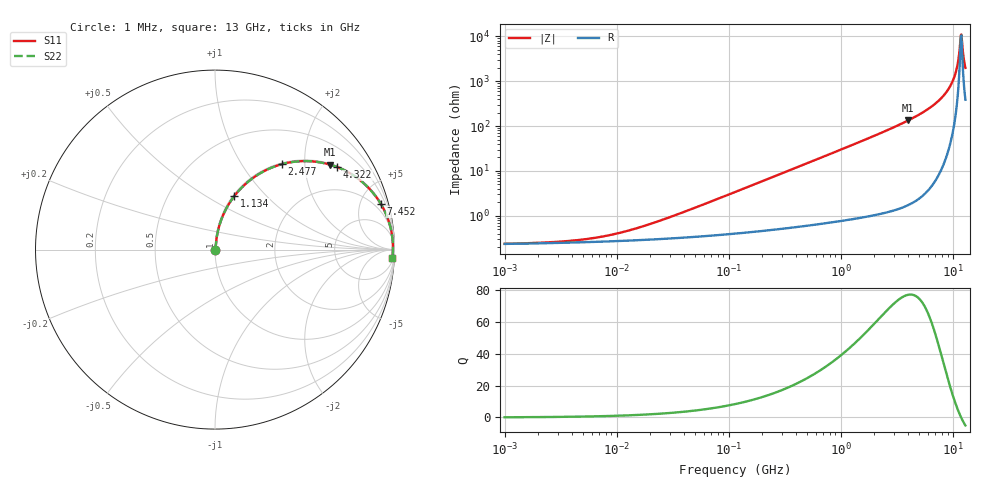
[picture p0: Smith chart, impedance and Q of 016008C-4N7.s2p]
# MHz S MA R 50
!Freq  MagS11  AngS11  MagS21  AngS21  MagS12  AngS12  MagS22  AngS22
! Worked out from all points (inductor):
!   801 points, 1 MHz to 13 GHz, reference 50 ohm
!   read as one part in series: L = 4.7 nH near 32.5 MHz
!   highest Q = 76.9 at 4.026 GHz (marker M1), where L = 5.31 nH
!   self-resonance near 11.83 GHz
!   S11 on the Smith chart (normalised r, x): 1 MHz: 1.00, +0.00; 1.134 GHz: 1.02, +0.68; 2.477 GHz: 1.02, +1.53; 4.322 GHz: 1.04, +2.94; 7.452 GHz: 1.16, +7.23; 13 GHz: 9, -39
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1  0.002383 7.1  0.9976 -0.0  0.9976 -0.0  0.002383 7.1
4.887486  0.002945 29.2  0.9974 -0.1  0.9974 -0.1  0.002945 29.2
10.428  0.004117 48.1  0.9973 -0.2  0.9973 -0.2  0.004117 48.1
23.60634  0.007577 66.1  0.997 -0.4  0.997 -0.4  0.007577 66.1
114.0175  0.03376 81.3  0.9954 -1.9  0.9954 -1.9  0.03376 81.3
557.2591  0.1619 78.5  0.9807 -9.3  0.9807 -9.3  0.1619 78.5
1133.974  0.3179 70.1  0.9406 -18.5  0.9406 -18.5  0.3179 70.1
1696.077  0.4519 62.1  0.8837 -26.9  0.8837 -26.9  0.4519 62.1
2477.441  0.6031 52.0  0.7886 -37.1  0.7886 -37.1  0.6031 52.0
2691.536  0.6376 49.6  0.7611 -39.6  0.7611 -39.6  0.6376 49.6
4025.713  0.797 36.4  0.5938 -52.8  0.5938 -52.8  0.797 36.4
4322.126  0.8219 34.0  0.5591 -55.3  0.5591 -55.3  0.8219 34.0
5880.315  0.9119 23.4  0.3971 -65.8  0.3971 -65.8  0.9119 23.4
7451.594  0.9585 15.4  0.2651 -73.4  0.2651 -73.4  0.9585 15.4
8899.91  0.9801 9.5  0.1648 -78.3  0.1648 -78.3  0.9801 9.5
10018.67  0.9882 5.6  0.09797 -80.3  0.09797 -80.3  0.9882 5.6
10756.34  0.9908 3.3  0.05808 -79.2  0.05808 -79.2  0.9908 3.3
11014.11  0.9912 2.5  0.0449 -77.5  0.0449 -77.5  0.9912 2.5
11548.33  0.9916 1.0  0.01936 -63.7  0.01936 -63.7  0.9916 1.0
11825.08  0.9915 0.2  0.009493 -25.8  0.009493 -25.8  0.9915 0.2
12252.68  0.9909 -0.9  0.0182 59.6  0.0182 59.6  0.9909 -0.9
13000  0.989 -2.8  0.05009 75.9  0.05009 75.9  0.989 -2.8
